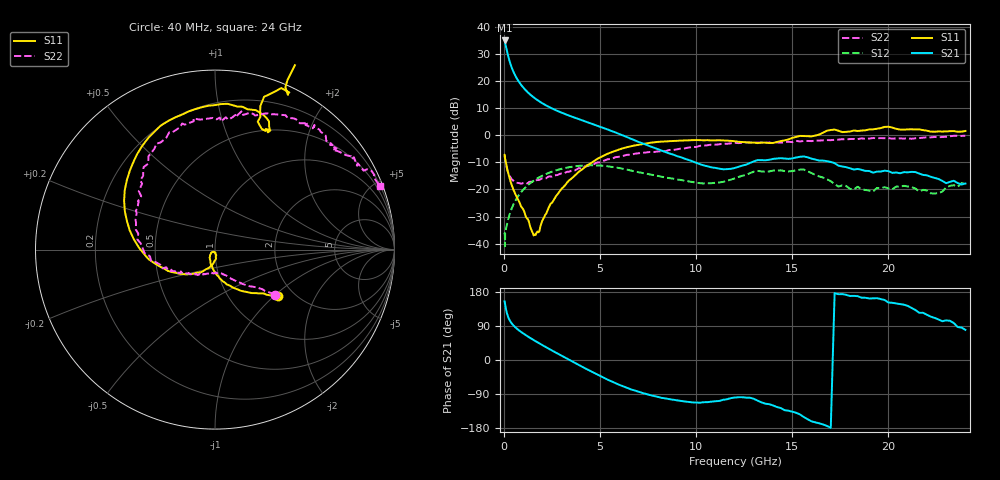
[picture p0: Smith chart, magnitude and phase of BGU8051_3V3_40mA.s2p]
! BGU8051_3V3_40mA
! Date/time Tue Jun 16 11:03:17 2015
! VAR V_out= 3.3000
! VAR I_out= 39.9550
! VAR V_in= 4.7320
! VAR I_in= 0.5544
# MHz S MA R 50
!  Freq-MHz  S11-mag  S11-arg  S21-mag  S21-arg  S12-mag  S12-arg  S22-mag  S22-arg
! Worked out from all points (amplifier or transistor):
!   187 points, 40 MHz to 24 GHz, reference 50 ohm
!   highest |S21| = 35.0 dB at 40 MHz (marker M1)
!   |S21| within 3 dB of that: start of sweep to 136.1 MHz
!   unconditionally stable (mu >= 1): 57.6 MHz to 61.86 MHz; 513.5 MHz to 13.17 GHz; 13.54 GHz to 13.72 GHz
!   at 750 MHz: K = 1.01, MAG = 20.5 dB, |S12| = -22.4 dB
!   at 5.4 GHz: K = 1.20, MAG = 4.1 dB, |S12| = -11.5 dB
!   at 24 GHz: K = 0.26, MSG = 0.1 dB, |S12| = -18.0 dB
!   lowest NFmin = 0.32 dB at 400 MHz
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40  0.4358 -36.3  56.08 154.7  0.01483 31.9  0.4175 -37.4
60  0.3817 -41.2  52.8 148.9  0.008986 30.4  0.3603 -39.6
80  0.352 -44.0  48.69 143.0  0.01651 36.6  0.3278 -41.1
120  0.2951 -53.2  42.11 132.3  0.01935 41.8  0.2799 -46.7
160  0.2527 -60.8  36.24 123.8  0.02258 48.8  0.2466 -51.0
200  0.2169 -67.7  31.44 117.1  0.0264 52.4  0.2203 -55.2
220  0.2044 -71.2  29.49 114.2  0.02754 53.8  0.2109 -56.2
280  0.1693 -78.6  24.5 107.1  0.0329 57.1  0.1863 -61.0
360  0.1356 -87.6  19.85 100.1  0.03991 59.6  0.1626 -65.1
440  0.1114 -94.7  16.61 94.6  0.04722 60.5  0.1505 -69.8
550  0.08977 -103.6  13.55 88.5  0.05738 60.5  0.1379 -74.4
700  0.06953 -111.7  10.79 81.7  0.07128 59.4  0.1322 -79.7
950  0.04591 -128.0  8.055 72.1  0.09382 56.0  0.1281 -89.0
1550  0.01419 -125.7  5.001 52.6  0.1448 44.5  0.1406 -108.2
2600  0.06416 -93.0  3.009 22.4  0.2188 21.4  0.1806 -130.0
4100  0.2384 -145.6  1.869 -18.6  0.2764 -12.9  0.2494 -151.3
6200  0.5757 151.6  0.9905 -69.5  0.2407 -55.3  0.4159 175.1
8200  0.763 109.8  0.5214 -99.8  0.1721 -75.3  0.5066 147.9
12200  0.7577 66.5  0.2611 -98.2  0.1695 -72.5  0.7163 103.6
16200  0.9866 66.6  0.3563 -164.6  0.1852 -148.8  0.7971 71.1
20200  1.385 32.4  0.2024 150.9  0.101 -147.3  0.8659 44.3
24000  1.198 20.1  0.1284 79.5  0.1254 -164.2  0.9837 21.2
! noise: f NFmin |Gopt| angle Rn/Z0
400  0.3232  0.1294  30.74  0.0498
550  0.3296  0.1028  41.09  0.0501
950  0.359  0.06365  91.53  0.0502
1250  0.393  0.07461  133.6  0.05
1600  0.4456  0.1066  159.9  0.0497
1900  0.5017  0.1356  172.8  0.0499
2250  0.58  0.1675  183.5  0.0509
2600  0.6723  0.1971  192.1  0.0533
3300  0.8985  0.2525  205.9  0.0639
4000  1.18  0.3063  216.5  0.0855
